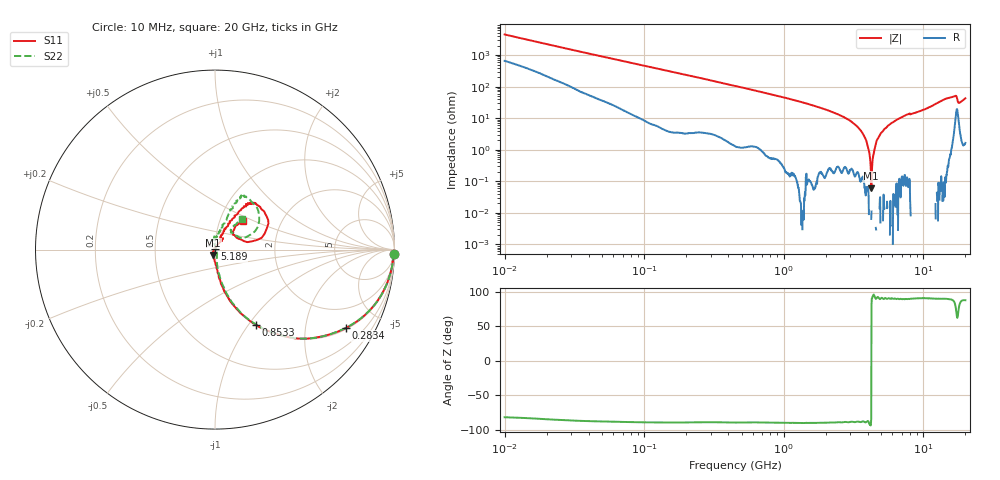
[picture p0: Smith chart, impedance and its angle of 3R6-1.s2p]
!Keysight Technologies,P5008B,MY61100088,A.16.20.02
!Date: Monday, May 27, 2024 15:15:03
!Correction: S11(C* 2-Port  )
!S21(C* 2-Port  )
!S12(C* 2-Port  )
!S22(C* 2-Port  )
!S2P File: Measurements: S11, S21, S12, S22:Log Frequency Sweep
# Hz S  dB  R 50
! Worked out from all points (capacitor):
!   1601 points, 10 MHz to 20 GHz, reference 50 ohm
!   read as one part in series: C = 3.6 pF near 10.39 MHz
!   lowest |Z| = 60.6 mohm at 4.23 GHz (marker M1)
!   series resonance near 4.24 GHz, so ESL is about 390 pH
!   S11 on the Smith chart (normalised r, x): 10 MHz: 7, -89; 283.4 MHz: 1.05, -3.31; 853.3 MHz: 1.00, -1.09; 5.189 GHz: 1.00, +0.01; 20 GHz: 1.28, +0.43
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1e7  -0.01 -1.3  -33.05 80.4  -33.05 80.4  -0.04 -1.3
3.555162e7  -0.06 -4.5  -22.03 82.4  -22.04 82.5  -0.07 -4.5
1.263918e8  -0.35 -15.2  -11.67 74.0  -11.68 74.0  -0.34 -15.2
2.834348e8  -1.40 -30.9  -5.84 58.0  -5.85 58.0  -1.41 -30.8
4.472136e8  -2.86 -43.5  -3.29 45.9  -3.30 45.9  -2.85 -43.4
8.533016e8  -6.42 -61.6  -1.16 28.0  -1.17 28.0  -6.42 -61.2
1.589917e9  -11.84 -76.1  -0.29 14.1  -0.30 14.1  -11.79 -75.0
2.976524e9  -19.85 -84.9  -0.03 3.8  -0.05 3.8  -20.01 -81.9
3.565405e9  -23.83 -92.0  -0.01 1.1  -0.02 1.1  -24.55 -80.6
4.230405e9  -29.91 -109.5  0.01 -1.5  0.00 -1.5  -31.08 -64.7
4.630008e9  -36.06 -128.2  0.01 -2.9  0.01 -2.9  -36.70 -47.0
5.019439e9  -42.54 -168.5  0.02 -4.1  0.01 -4.1  -43.73 -10.3
5.189161e9  -47.50 118.7  0.02 -4.6  0.01 -4.6  -41.88 24.3
5.313894e9  -41.86 113.5  0.02 -5.0  0.01 -5.0  -41.47 57.4
5.652411e9  -35.42 79.6  0.02 -5.9  0.01 -5.9  -35.70 85.8
6.275133e9  -28.99 63.4  0.02 -7.6  0.01 -7.6  -29.53 95.4
7.236311e9  -24.22 51.7  0.02 -10.2  0.00 -10.1  -24.77 98.9
9.622897e9  -23.04 64.1  0.03 -15.9  0.02 -15.9  -22.75 83.7
1.447892e10  -10.26 55.9  -0.37 -28.7  -0.38 -28.7  -10.20 64.3
1.67762e10  -9.24 38.9  -0.91 -34.5  -0.92 -34.5  -9.48 53.3
1.836088e10  -17.72 40.2  -0.29 -29.7  -0.30 -29.7  -17.78 46.9
2e10  -13.05 46.2  -0.30 -37.1  -0.31 -37.1  -12.88 48.5
